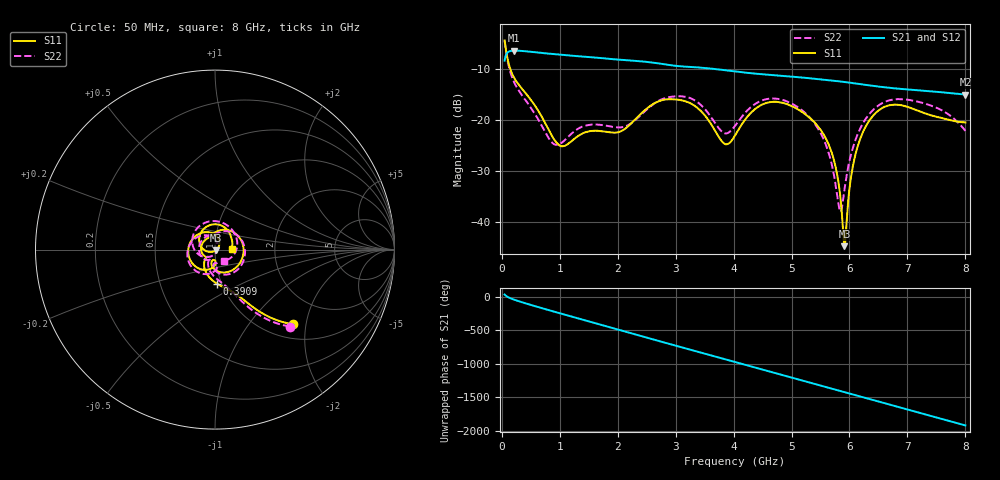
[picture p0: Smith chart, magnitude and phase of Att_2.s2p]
#  HZ  S  DB  R  50.00
! Rohde & Schwarz Vector Network Analyzer
! Rohde-Schwarz,ZNB40-4Port,1311601084101679,3.45
! Created: UTC 4/25/2025, 9:29:20 AM
! freq[Hz]  db:S11  ang:S11  db:S21  ang:S21  db:S12  ang:S12  db:S22  ang:S22
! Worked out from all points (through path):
!   1750 points, 50 MHz to 8 GHz, reference 50 ohm
!   highest |S21| = -6.40 dB at 213.6 MHz (marker M1); lowest = -15.0 dB at 8 GHz (marker M2)
!   group delay of S21, straight-line fit = 667 ps
!   lowest |S11| = -44.8 dB at 5.914 GHz (marker M3), VSWR 1.01, Z = 50.3 - j0.465 ohm
!   |S11| at or under -10 dB: 147.5 MHz to end of sweep
!   |S22| runs from -38.0 to -4.5 dB; largest |S21 - S12| = 0.00054
!   S11 on the Smith chart (normalised r, x): 50 MHz: 1.30, -1.69; 390.9 MHz: 0.95, -0.37; 8 GHz: 1.21, +0.00
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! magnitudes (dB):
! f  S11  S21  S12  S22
! 50 MHz  -4.4  -8.4  -8.4  -4.5
! 213.6 MHz  -11.7  -6.4  -6.4  -12.6
! 390.9 MHz  -14.5  -6.5  -6.5  -15.8
! 909.1 MHz  -23.9  -7.1  -7.1  -24.8
! 1.377 GHz  -22.8  -7.6  -7.6  -21.4
! 2.127 GHz  -21.8  -8.3  -8.3  -21.3
! 2.7 GHz  -16.4  -8.9  -8.9  -16.3
! 3.227 GHz  -16.6  -9.6  -9.6  -15.6
! 3.836 GHz  -24.6  -10.2  -10.2  -22.6
! 4.027 GHz  -23.0  -10.5  -10.5  -21.1
! 4.605 GHz  -16.6  -11.1  -11.1  -15.9
! 5.35 GHz  -19.9  -11.9  -11.9  -20.0
! 5.568 GHz  -23.1  -12.1  -12.1  -24.2
! 5.723 GHz  -27.5  -12.3  -12.3  -30.2
! 5.836 GHz  -34.5  -12.5  -12.5  -37.9
! 5.914 GHz  -44.8  -12.6  -12.6  -33.7
! 6.036 GHz  -30.5  -12.7  -12.7  -26.4
! 6.168 GHz  -24.3  -12.9  -12.9  -22.1
! 6.386 GHz  -19.5  -13.3  -13.3  -18.3
! 6.677 GHz  -17.2  -13.7  -13.7  -16.2
! 7.468 GHz  -19.3  -14.4  -14.5  -17.5
! 8 GHz  -20.5  -15.0  -15.0  -22.1
